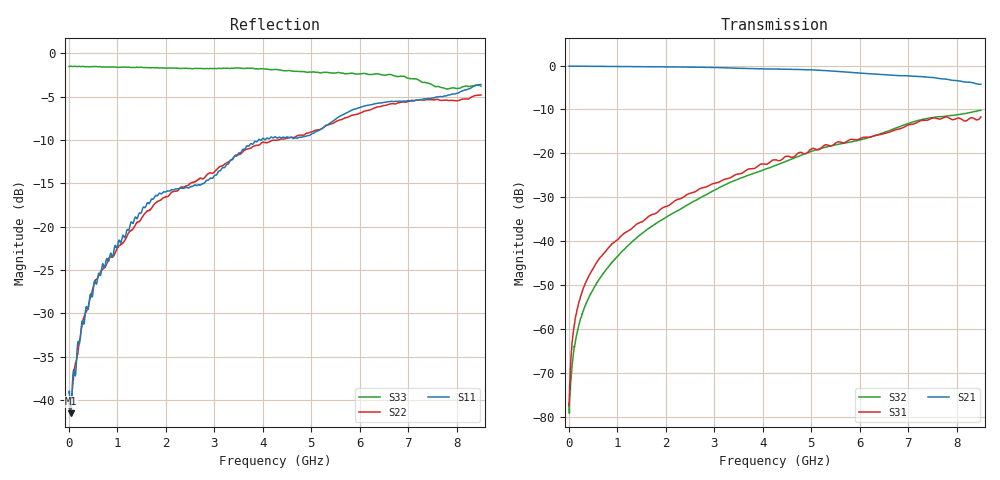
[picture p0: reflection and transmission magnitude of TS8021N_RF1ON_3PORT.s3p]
!Created with skrf (http://scikit-rf.org).
# GHz S RI R 50.0
!freq ReS11 ImS11 ReS12 ImS12 ReS13 ImS13
! ReS21 ImS21 ReS22 ImS22 ReS23 ImS23
! ReS31 ImS31 ReS32 ImS32 ReS33 ImS33
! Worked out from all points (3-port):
!   1601 points, 10 MHz to 8.5 GHz, reference 50 ohm
!   strongest paths, dB at 10 MHz, 2.132 GHz, 4.255 GHz, 6.378 GHz, 8.5 GHz:
!     S21: -0.1, -0.3, -0.8, -2.0, -4.3
!     S31: -77.4, -31.3, -21.5, -15.8, -11.7
!     S32: -76.8, -33.8, -22.8, -15.8, -10.2
!   lowest |S11| = -41.5 dB at 41.84 MHz (marker M1), VSWR 1.02, Z = 50.7 - j0.482 ohm
!   |S11| at or under -10 dB: start of sweep to 3.912 GHz; 3.946 GHz to 3.976 GHz (29.46 MHz wide, 0.744 % of centre)
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0.01  0.011 0.000603  0.9849 -0.00296  0.000115 9.91e-05
      0.9849 -0.00308  0.0095 0.000616  7.63e-05 5.76e-05
      7.21e-05 0.000114  0.000129 6.34e-05  -0.838 0.00262
0.0418375  0.00691 -0.00475  0.985 -0.0124  9.35e-05 0.000396
           0.9848 -0.012  0.0083 -0.00335  9.27e-05 0.000198
           0.000111 0.000419  8.76e-05 0.000232  -0.8415 0.00757
0.1108187  0.00797 -0.0123  0.9839 -0.0322  9.06e-05 0.00104
           0.984 -0.0324  0.00898 -0.0113  6.85e-05 0.000581
           9.4e-05 0.00105  5.8e-05 0.000587  -0.8397 0.0192
0.2700063  0.00779 -0.0267  0.9803 -0.0782  -4.98e-05 0.00256
           0.9804 -0.0783  0.00767 -0.0251  -8.49e-05 0.00143
           -3.38e-05 0.00255  -5.82e-05 0.0014  -0.8361 0.0462
0.8696125  -0.0103 -0.0696  0.9475 -0.2446  -0.000911 0.00898
           0.9476 -0.2444  -0.012 -0.066  -0.00138 0.00537
           -0.000941 0.00896  -0.00139 0.00537  -0.8148 0.1738
1.819431  -0.0522 -0.1416  0.8362 -0.4881  -0.00302 0.021
          0.8361 -0.4883  -0.0783 -0.1147  -0.00373 0.0157
          -0.00297 0.021  -0.00372 0.0157  -0.7507 0.3427
4.255  -0.304 -0.1271  0.2938 -0.8646  0.0203 0.082
       0.293 -0.8636  -0.3029 -0.0853  0.02 0.0696
       0.0203 0.0818  0.0201 0.0698  -0.4282 0.6813
6.388113  -0.4884 0.167  -0.263 -0.749  0.1112 0.1192
          -0.2631 -0.7489  -0.4453 0.2069  0.1339 0.0946
          0.1112 0.1192  0.1341 0.0944  -6.89e-06 0.7586
7.237113  -0.4693 0.2661  -0.408 -0.6315  0.1944 0.1283
          -0.4089 -0.6312  -0.3391 0.4148  0.2299 0.065
          0.1946 0.128  0.2303 0.0653  0.0695 0.6912
8.5  -0.2939 0.5908  -0.5019 -0.3485  0.2525 0.0619
     -0.5025 -0.349  -0.141 0.5564  0.3021 -0.0717
     0.2527 0.0621  0.3022 -0.0718  0.3911 0.5132
